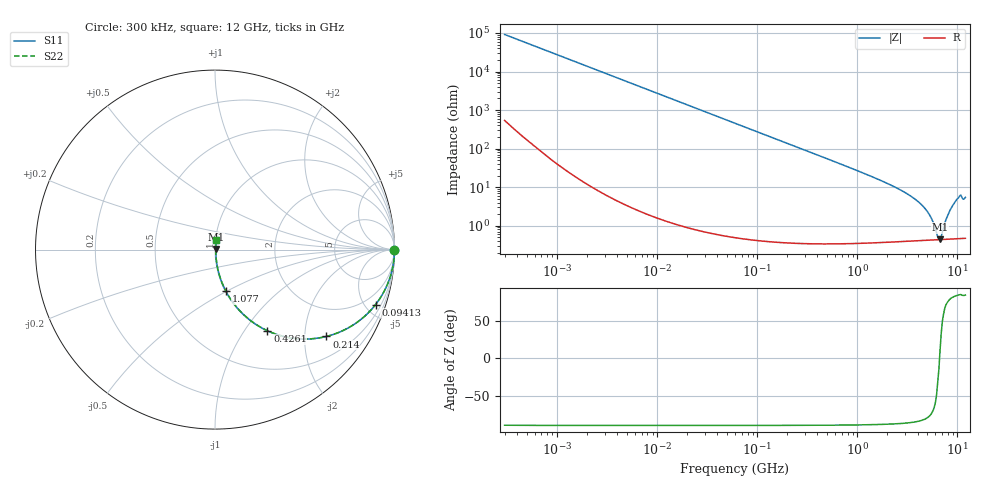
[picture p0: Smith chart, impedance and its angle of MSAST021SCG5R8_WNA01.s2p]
! MSAST021SCG5R8_WNA01  S-PARAMETER MODEL  ( General Type )
! Model Generated by TAIYO YUDEN Corporation (http://www.ty-top.com)
! Version 2.0
! TAIYO YUDEN Control No. 181101
! Copyright(c) 2015 TAIYO YUDEN CO.,LTD. All Rights Reserved.
! Product Description (link to TY-COMPAS)
! https://ds.yuden.co.jp/TYCOMPAS/or/detail?pn=MSAST021SCG5R8CWNA01&u=M
! Products Name : Multilayer Ceramic Capacitors
! Characteristics :
!  Capacitance : 5.8 pF , Rated Voltage : 25V , TCC : CG / C0G
!  Case Size : 0.25 x 0.125 / 0.0098 x 0.0049 [mm/inch] , Thickness : 0.125 / 0.0049 [mm/inch]
!  (Conditions: Temperature = 25 degC , DC Bias Current/Voltage = 0A / 0V)
! External Node Assignments :
!  1  o---| |---o  2
! GND o---------o GND
! Frequency Range : 0.3MHz  -  12000MHz  [ 401 STEP ]
# MHz S RI R 50
! Freq[MHz].  S11 Real  S11 Imag  S21 Real  S21 Imag  S12 Real  S12 Imag  S22 Real  S22 Imag
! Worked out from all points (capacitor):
!   401 points, 300 kHz to 12 GHz, reference 50 ohm
!   read as one part in series: C = 5.8 pF near 316.3 kHz
!   lowest |Z| = 445 mohm at 6.7 GHz (marker M1)
!   series resonance near 6.624 GHz, so ESL is about 100 pH
!   S11 on the Smith chart (normalised r, x): 300 kHz: open; 94.13 MHz: 1.01, -5.83; 214 MHz: 1.01, -2.56; 426.1 MHz: 1.01, -1.28; 1.077 GHz: 1.01, -0.50; 12 GHz: 1.01, +0.11
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0.3  1 -0.00109  7.64e-06 0.00109  7.64e-06 0.00109  1 -0.00109
1.769972  1 -0.00645  4.76e-05 0.00645  4.76e-05 0.00645  1 -0.00645
10.44266  0.9985 -0.038  0.00147 0.038  0.00147 0.038  0.9985 -0.038
60  0.9542 -0.2086  0.0458 0.2086  0.0458 0.2086  0.9542 -0.2086
94.13233  0.8943 -0.3067  0.1057 0.3067  0.1057 0.3067  0.8943 -0.3067
213.9924  0.621 -0.4838  0.379 0.4838  0.379 0.4838  0.621 -0.4838
353.9943  0.3745 -0.4818  0.6255 0.4818  0.6255 0.4818  0.3745 -0.4818
426.1204  0.2924 -0.4522  0.7076 0.4522  0.7076 0.4522  0.2924 -0.4522
668.5285  0.1437 -0.3467  0.8563 0.3467  0.8563 0.3467  0.1437 -0.3467
1076.992  0.0608 -0.232  0.9392 0.232  0.9392 0.232  0.0608 -0.232
2088.533  0.0173 -0.1156  0.9827 0.1156  0.9827 0.1156  0.0173 -0.1156
3276.641  0.00784 -0.0621  0.9922 0.0621  0.9922 0.0621  0.00784 -0.0621
4502.883  0.00515 -0.0319  0.9948 0.0319  0.9948 0.0319  0.00515 -0.0319
5278.635  0.00455 -0.0182  0.9955 0.0182  0.9955 0.0182  0.00455 -0.0182
5715.274  0.00439 -0.0115  0.9956 0.0115  0.9956 0.0115  0.00439 -0.0115
6354.153  0.00433 -0.00267  0.9957 0.00267  0.9957 0.00267  0.00433 -0.00267
6699.894  0.00435 0.000852  0.9956 -0.000852  0.9956 -0.000852  0.00435 0.000852
7064.448  0.00441 0.00513  0.9956 -0.00513  0.9956 -0.00513  0.00441 0.00513
8064.993  0.00481 0.0187  0.9952 -0.0187  0.9952 -0.0187  0.00481 0.0187
9207.246  0.00588 0.0365  0.9941 -0.0365  0.9941 -0.0365  0.00588 0.0365
10511.28  0.00803 0.0582  0.992 -0.0582  0.992 -0.0582  0.00803 0.0582
12000  0.00758 0.0536  0.9924 -0.0536  0.9924 -0.0536  0.00758 0.0536
